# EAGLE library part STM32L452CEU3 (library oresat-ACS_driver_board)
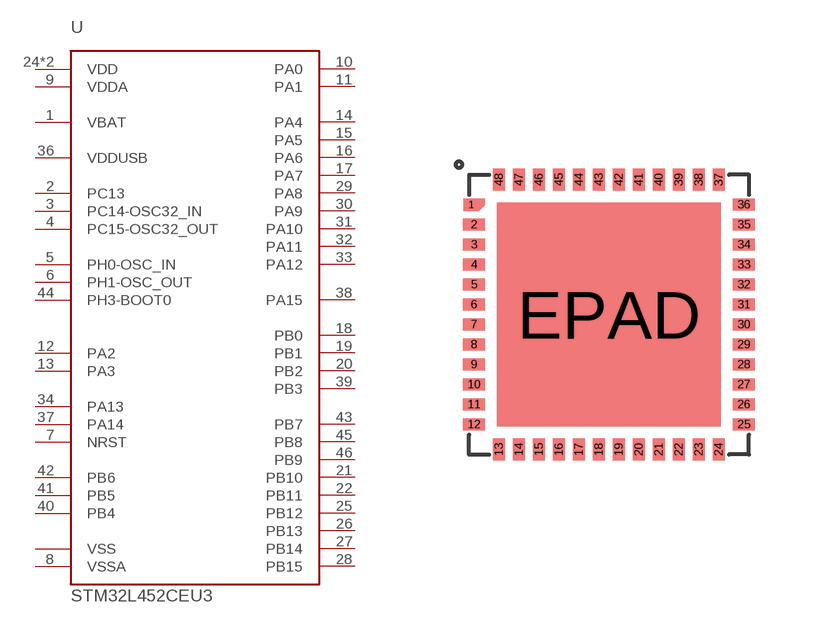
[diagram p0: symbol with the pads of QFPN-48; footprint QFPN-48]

Designator prefix -

## STM32L452CEU3  [QFPN-48]
1  VBAT
2  PC13
3  PC14-OSC32_IN
4  PC15-OSC32_OUT
5  PH0-OSC_IN
6  PH1-OSC_OUT
7  NRST
8  VSSA
9  VDDA
10  PA0
11  PA1
12  PA2
13  PA3
14  PA4
15  PA5
16  PA6
17  PA7
18  PB0
19  PB1
20  PB2
21  PB10
22  PB11
23  VSS
24  VDD
25  PB12
26  PB13
27  PB14
28  PB15
29  PA8
30  PA9
31  PA10
32  PA11
33  PA12
34  PA13
35  VSS
36  VDDUSB
37  PA14
38  PA15
39  PB3
40  PB4
41  PB5
42  PB6
43  PB7
44  PH3-BOOT0
45  PB8
46  PB9
47  VSS
48  VDD
EPAD  VSS

## Footprint QFPN-48 (pad centres in mm)
smd 0.38 x 0.28: 1 -3.45,2.75
smd 0.55 x 0.3: 2 -3.375,2.25; 3 -3.375,1.75; 4 -3.375,1.25; 5 -3.375,0.75; 6 -3.375,0.25; 7 -3.375,-0.25; 8 -3.375,-0.75; 9 -3.375,-1.25; 10 -3.375,-1.75; 11 -3.375,-2.25; 12 -3.375,-2.75; 25 3.375,-2.75; 26 3.375,-2.25; 27 3.375,-1.75; 28 3.375,-1.25; 29 3.375,-0.75; 30 3.375,-0.25; 31 3.375,0.25; 32 3.375,0.75; 33 3.375,1.25; 34 3.375,1.75; 35 3.375,2.25; 36 3.375,2.75
smd 0.3 x 0.55: 13 -2.75,-3.375; 14 -2.25,-3.375; 15 -1.75,-3.375; 16 -1.25,-3.375; 17 -0.75,-3.375; 18 -0.25,-3.375; 19 0.25,-3.375; 20 0.75,-3.375; 21 1.25,-3.375; 22 1.75,-3.375; 23 2.25,-3.375; 24 2.75,-3.375; 37 2.75,3.375; 38 2.25,3.375; 39 1.75,3.375; 40 1.25,3.375; 41 0.75,3.375; 42 0.25,3.375; 43 -0.25,3.375; 44 -0.75,3.375; 45 -1.25,3.375; 46 -1.75,3.375; 47 -2.25,3.375; 48 -2.75,3.375
smd 5.6 x 5.6: EPAD 0,0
